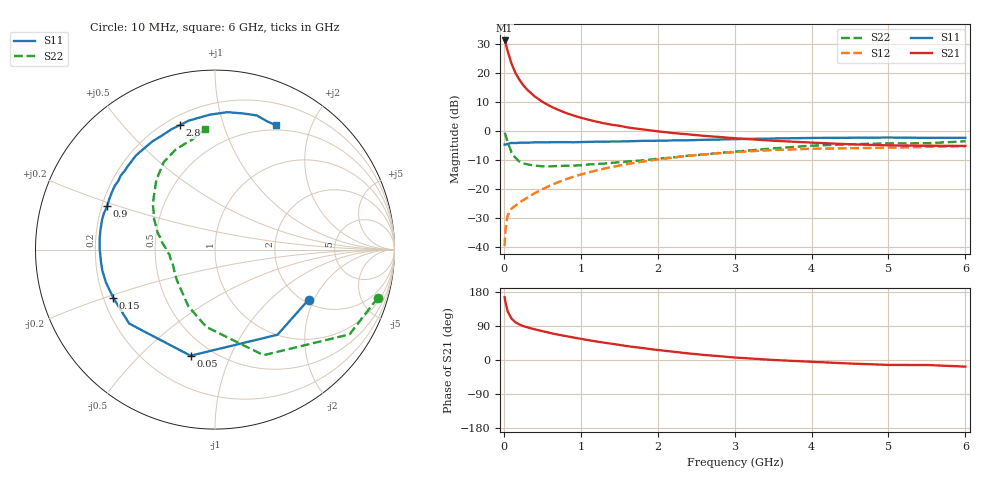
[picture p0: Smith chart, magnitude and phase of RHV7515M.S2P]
! SIEMENS Small Signal Semiconductors
! BFR106
! Si NPN RF Bipolar Junction Transistor in SOT23
! VCE = 0.75 V  IC = 15 mA
! Common Emitter S-Parameters:  August  1996
# GHz  S  MA  R  50
!  f  S11  S21  S12  S22
! GHz  MAG  ANG  MAG  ANG  MAG  ANG  MAG  ANG
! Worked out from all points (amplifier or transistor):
!   36 points, 10 MHz to 6 GHz, reference 50 ohm
!   highest |S21| = 31.4 dB at 10 MHz (marker M1)
!   |S21| within 3 dB of that: start of sweep to 43.06 MHz
!   unconditionally stable (mu >= 1): 373.7 MHz to end of sweep
!   at 250 MHz: K = 0.86, MSG = 19.9 dB, |S12| = -23.8 dB
!   at 1.4 GHz: K = 1.11, MAG = 5.3 dB, |S12| = -12.3 dB
!   at 6 GHz: K = 1.03, MAG = -1.0 dB, |S12| = -5.1 dB
!   S11 on the Smith chart (normalised r, x): 10 MHz: 2.12, -1.82; 50 MHz: 0.39, -0.72; 150 MHz: 0.24, -0.21; 900 MHz: 0.22, +0.18; 2.8 GHz: 0.25, +0.73; 6 GHz: 0.44, +1.51
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0.01  0.5914 -28.2  37.08 165.5  0.0104 79.9  0.9458 -16.5
0.02  0.5885 -53.7  34.36 153.4  0.0195 68.9  0.8861 -32.2
0.05  0.6067 -103.0  24.21 128.0  0.0355 50.5  0.6476 -65.3
0.1  0.6312 -139.2  14.75 109.0  0.0463 42.1  0.4333 -96.5
0.15  0.6273 -154.7  10.23 99.7  0.0521 43.0  0.349 -115.2
0.2  0.6346 -163.2  7.848 94.0  0.0583 45.6  0.3027 -126.6
0.25  0.6385 -169.6  6.306 89.6  0.0646 48.2  0.28 -136.6
0.3  0.6389 -173.7  5.293 86.5  0.0709 51.0  0.2697 -142.8
0.4  0.643 179.3  4.023 81.0  0.0854 54.5  0.2558 -152.5
0.5  0.6459 174.3  3.24 76.2  0.1 56.7  0.2495 -159.1
0.6  0.6479 169.7  2.728 71.5  0.1154 57.9  0.2486 -163.3
0.7  0.6506 165.4  2.372 67.0  0.1314 58.2  0.2522 -167.0
0.9  0.6474 158.1  1.885 59.5  0.1637 57.8  0.2547 -173.5
1.1  0.6572 151.0  1.588 52.3  0.1949 56.2  0.2674 -177.8
1.3  0.6606 144.6  1.379 45.8  0.2266 53.9  0.2775 177.4
1.6  0.6726 136.1  1.174 36.7  0.2711 49.9  0.3005 171.3
2.2  0.6963 120.2  0.934 21.9  0.353 40.5  0.3535 158.3
2.8  0.7208 105.7  0.799 10.1  0.4185 30.5  0.4241 144.6
3.5  0.7521 92.3  0.688 0.1  0.4751 19.5  0.5067 130.2
4.5  0.7746 78.4  0.598 -9.3  0.5116 5.2  0.5985 111.5
5.5  0.771 67.6  0.565 -13.2  0.5374 -3.4  0.6231 102.3
6  0.7717 63.8  0.56 -17.5  0.5538 -9.7  0.6724 94.8
